|-- THIS SOFTWARE IS PROVIDED BY FREESCALE "AS IS" AND ANY EXPRESSED OR
|-- IMPLIED WARRANTIES, INCLUDING, BUT NOT LIMITED TO, THE IMPLIED WARRANTIES
|-- OF MERCHANTABILITY AND FITNESS FOR A PARTICULAR PURPOSE ARE DISCLAIMED.
|-- IN NO EVENT SHALL FREESCALE OR ITS CONTRIBUTORS BE LIABLE FOR ANY DIRECT,
|-- INDIRECT, INCIDENTAL, SPECIAL, EXEMPLARY, OR CONSEQUENTIAL DAMAGES
|-- (INCLUDING, BUT NOT LIMITED TO, PROCUREMENT OF SUBSTITUTE GOODS OR
|-- SERVICES; LOSS OF USE, DATA, OR PROFITS; OR BUSINESS INTERRUPTION)
|-- HOWEVER CAUSED AND ON ANY THEORY OF LIABILITY, WHETHER IN CONTRACT,
|-- STRICT LIABILITY, OR TORT (INCLUDING NEGLIGENCE OR OTHERWISE) ARISING
|-- IN ANY WAY OUT OF THE USE OF THIS SOFTWARE, EVEN IF ADVISED OF
|-- THE POSSIBILITY OF SUCH DAMAGE.
[IBIS Ver]   5.0
[Comment Char] |_char
[File name]   k60_120_144lqfp_full.ibs
[File Rev]   1.2
[Date]   12/03/2013
[Source]   Freescale, MSG, MCD, Design
[Notes]   IBIS model for K60 microprocessor covers 1.71 - 3.6V range
[Disclaimer]   The model given below represents 144LQFP package on K60 family
[Copyright]   Copyright, Freescale, Inc., 2013
|  Component K60
[Component]   K60
[Manufacturer]  Freescale, Inc.
[Package]
|   typ   min   max
R_pkg   0.13643   0.074674   0.1605
L_pkg   6.219e-9   4.626e-9   7.688e-9
C_pkg   1.386e-12   1.181e-12   1.778e-12
[Pin]   Signal_name   model_name   R_pin   L_pin   C_pin
31   VDDA   POWER
5   VDD   POWER
16   VDD   POWER
43   VDD   POWER
56   VDD   POWER
70   VDD   POWER
94   VDD   POWER
108   VDD   POWER
122   VDD   POWER
135   VDD   POWER
42   VBAT   POWER
21   VOUT33   POWER
22   VREGIN   POWER
36   ADC0SE16   NC   0.14655   6.97e-9   1.242e-12
35   ADC1SE16   NC   0.15005   5.832e-9   1.506e-12
38   DAC0OUT   NC   0.14297   7.255e-9   1.542e-12
39   DAC1OUT   NC   0.14077   7.112e-9   1.559e-12
41   EXTAL32   NC   0.15038   6.782e-9   1.534e-12
28   PGA0DM   NC   0.12334   5.949e-9   1.339e-12
27   PGA0DP   NC   0.12106   5.958e-9   1.357e-12
30   PGA1DM   NC   0.13667   5.32e-9   1.386e-12
29   PGA1DP   NC   0.12773   5.801e-9   1.374e-12
24   PGA2DM   NC   0.11967   5.705e-9   1.317e-12
23   PGA2DP   NC   0.12104   5.634e-9   1.22e-12
26   PGA3DM   NC   0.11999   5.914e-9   1.36e-12
25   PGA3DP   NC   0.11921   5.753e-9   1.321e-12
50   PTA0   io_5vtol   0.14193   6.304e-9   1.346e-12
51   PTA1   io_5vtol   0.14175   6.208e-9   1.311e-12
52   PTA2   io_5vtol   0.14204   6.057e-9   1.268e-12
53   PTA3   io_5vtol   0.14336   5.897e-9   1.296e-12
54   PTA4   io_5vtol   0.14599   5.67e-9   1.273e-12
55   PTA5   io_5vtol   0.15141   5.209e-9   1.264e-12
58   PTA6   io_fast_5vtol   0.14704   5.445e-9   1.181e-12
59   PTA7   io_fast_5vtol   0.14318   5.955e-9   1.316e-12
60   PTA8   io_fast_5vtol   0.14221   6.155e-9   1.403e-12
61   PTA9   io_fast_5vtol   0.14262   6.348e-9   1.365e-12
62   PTA10   io_fast_5vtol   0.14414   6.614e-9   1.329e-12
63   PTA11   io_fast_5vtol   0.14519   6.744e-9   1.315e-12
64   PTA12   io_fast_5vtol   0.14748   6.905e-9   1.497e-12
65   PTA13   io_fast_5vtol   0.15026   7.017e-9   1.504e-12
66   PTA14   io_fast_5vtol   0.15364   7.127e-9   1.546e-12
67   PTA15   io_fast_5vtol   0.15784   7.187e-9   1.595e-12
68   PTA16   io_fast_5vtol   0.15454   6.819e-9   1.507e-12
69   PTA17   io_fast_5vtol   0.16279   6.406e-9   1.497e-12
72   PTA18   io_5vtol   0.16043   6.526e-9   1.251e-12
73   PTA19   io_5vtol   0.15124   7.53e-9   1.238e-12
75   PTA24   io_fast_5vtol   0.14588   7.278e-9   1.672e-12
76   PTA25   io_fast_5vtol   0.14088   7.144e-9   1.574e-12
77   PTA26   io_fast_5vtol   0.13659   6.98e-9   1.557e-12
78   PTA27   io_fast_5vtol   0.13268   6.792e-9   1.527e-12
79   PTA28   io_fast_5vtol   0.12945   6.656e-9   1.373e-12
80   PTA29   io_fast_5vtol   0.12683   6.534e-9   1.39e-12
81   PTB0   io_5vtol   0.12814   6.465e-9   1.315e-12
82   PTB1   io_5vtol   0.12562   6.334e-9   1.282e-12
83   PTB2   io_5vtol   0.12444   6.322e-9   1.332e-12
84   PTB3   io_5vtol   0.12222   6.072e-9   1.188e-12
85   PTB4   io_5vtol   0.12112   5.946e-9   1.208e-12
86   PTB5   io_5vtol   0.12035   5.788e-9   1.261e-12
87   PTB6   io_5vtol   0.1205   5.733e-9   1.251e-12
88   PTB7   io_5vtol   0.12088   5.617e-9   1.323e-12
89   PTB8   io_5vtol   0.12212   5.499e-9   1.25e-12
90   PTB9   io_5vtol   0.12418   5.384e-9   1.259e-12
91   PTB10   io_5vtol   0.12712   5.169e-9   1.236e-12
92   PTB11   io_5vtol   0.13355   4.626e-9   1.199e-12
95   PTB16   io_5vtol   0.1273   5.128e-9   1.245e-12
96   PTB17   io_5vtol   0.12586   5.485e-9   1.249e-12
97   PTB18   io_5vtol   0.12629   5.716e-9   1.269e-12
98   PTB19   io_5vtol   0.12517   6.017e-9   1.309e-12
99   PTB20   io_5vtol   0.12713   6.21e-9   1.298e-12
100   PTB21   io_5vtol   0.12288   6.219e-9   1.481e-12
101   PTB22   io_5vtol   0.12499   6.323e-9   1.434e-12
102   PTB23   io_5vtol   0.12787   6.437e-9   1.509e-12
103   PTC0   io_5vtol   0.1316   6.547e-9   1.606e-12
104   PTC1   io_5vtol   0.1361   6.536e-9   1.477e-12
105   PTC2   io_5vtol   0.14259   6.455e-9   1.623e-12
106   PTC3   io_5vtol   0.1535   5.859e-9   1.717e-12
109   PTC4   io_5vtol   0.15098   7.253e-9   1.234e-12
110   PTC5   io_5vtol   0.14677   7.215e-9   1.63e-12
111   PTC6   io_5vtol   0.14359   7.131e-9   1.778e-12
112   PTC7   io_5vtol   0.14177   7.069e-9   1.644e-12
113   PTC8   io_5vtol   0.14008   6.972e-9   1.555e-12
114   PTC9   io_5vtol   0.1389   6.86e-9   1.458e-12
115   PTC10   io_5vtol   0.13814   6.784e-9   1.455e-12
116   PTC11   io_5vtol   0.14256   6.761e-9   1.421e-12
117   PTC12   io_5vtol   0.14197   6.609e-9   1.445e-12
118   PTC13   io_5vtol   0.14182   6.363e-9   1.338e-12
119   PTC14   io_5vtol   0.14393   6.114e-9   1.299e-12
120   PTC15   io_5vtol   0.15069   5.442e-9   1.29e-12
123   PTC16   io_5vtol   0.15095   5.346e-9   1.331e-12
124   PTC17   io_5vtol   0.14574   5.72e-9   1.254e-12
125   PTC18   io_5vtol   0.14294   5.845e-9   1.28e-12
126   PTC19   io_5vtol   0.1425   5.923e-9   1.323e-12
127   PTD0   io_5vtol   0.14188   5.956e-9   1.311e-12
128   PTD1   io_5vtol   0.14138   5.999e-9   1.364e-12
129   PTD2   io_5vtol   0.14138   6.02e-9   1.256e-12
130   PTD3   io_5vtol   0.14182   6.003e-9   1.269e-12
131   PTD4   io_5vtol   0.14319   5.979e-9   1.332e-12
132   PTD5   io_5vtol   0.14586   5.856e-9   1.384e-12
133   PTD6   io_5vtol   0.1519   5.479e-9   1.337e-12
136   PTD7   io_5vtol   0.095186   5.041e-9   1.478e-12
137   PTD8   io_5vtol   0.14925   6.316e-9   1.492e-12
138   PTD9   io_5vtol   0.14703   6.779e-9   1.509e-12
139   PTD10   io_5vtol   0.14768   7.034e-9   1.474e-12
140   PTD11   io_5vtol   0.14919   7.21e-9   1.461e-12
141   PTD12   io_5vtol   0.14283   7.2e-9   1.515e-12
142   PTD13   io_5vtol   0.1446   7.355e-9   1.608e-12
143   PTD14   io_5vtol   0.14714   7.47e-9   1.636e-12
144   PTD15   io_5vtol   0.15009   7.688e-9   1.254e-12
1   PTE0   io_5vtol   0.1427   7.238e-9   1.207e-12
2   PTE1   io_5vtol   0.13901   6.841e-9   1.585e-12
3   PTE2   io_5vtol   0.1373   6.39e-9   1.599e-12
4   PTE3   io_5vtol   0.14055   5.484e-9   1.55e-12
7   PTE4   io_5vtol   0.13988   5.539e-9   1.415e-12
8   PTE5   io_5vtol   0.13191   5.975e-9   1.399e-12
9   PTE6   io_5vtol   0.12792   6.051e-9   1.458e-12
10   PTE7   io_5vtol   0.128   6.113e-9   1.36e-12
11   PTE8   io_5vtol   0.12596   6.019e-9   1.327e-12
12   PTE9   io_5vtol   0.12369   5.831e-9   1.207e-12
13   PTE10   io_5vtol   0.12287   5.649e-9   1.215e-12
14   PTE11   io_5vtol   0.12314   5.391e-9   1.263e-12
15   PTE12   io_5vtol   0.1281   4.876e-9   1.189e-12
45   PTE24   io_5vtol   0.1605   5.873e-9   1.334e-12
46   PTE25   io_5vtol   0.152   6.343e-9   1.407e-12
47   PTE26   io_5vtol   0.14753   6.409e-9   1.316e-12
48   PTE27   io_5vtol   0.14454   6.387e-9   1.329e-12
49   PTE28   io_5vtol   0.14278   6.348e-9   1.243e-12
74   RESETB   io_5vtol   0.089297   6.831e-9   1.632e-12
20   USB0DM   NC   0.12719   5.235e-9   1.265e-12
19   USB0DP   NC   0.13445   4.892e-9   1.192e-12
32   VREFH   NC   0.14189   5.271e-9   1.448e-12
33   VREFL   NC   0.14543   5.412e-9   1.448e-12
37   VREFOUT   NC   0.14666   7.499e-9   1.204e-12
40   XTAL32   NC   0.15094   7.153e-9   1.538e-12
34   VSSA   GND
6   VSS   GND
17   VSS   GND
18   VSS   GND
44   VSS   GND
57   VSS   GND
71   VSS   GND
93   VSS   GND
107   VSS   GND
121   VSS   GND
134   VSS   GND
|End [Component]
[Component] io80u65dgo6m5vtol
|   Component io80u65dgo6m5vtol
| This component was characterised for following simulation conditions:
| Temperature:
|   - Typ: 25.0C,   - Min: 125.0C,   - Max: -40.0C
| External (pad) voltage:
|   - Typ: 3.3V,   - Min: 1.71V,   - Max: 3.6V
| Internal (core) voltage:
|   - Typ: 1.2V,   - Min: 1.08V,   - Max: 1.32V
[Manufacturer] Freescale Semiconductor
[Package]
| variable   typ   min   max
R_pkg   0.2240   0.2240   0.2240
L_pkg   8.5100nH   8.5100nH   8.5100nH
C_pkg   0.2740pF   0.2740pF   0.2740pF
[Pin]  signal_name   model_name   R_pin   L_pin   C_pin
fpad   pad   io_fast_5vtol
pad   pad   io_5vtol
|vsslv vsslv   iGND
|vddlv vddlv   iPOWER
vdd3v  vdd3v   POWER
vss3v  vss3v   GND
|obe   obe   dummy
|do   do   dummy
[Model Selector] io_fast_5vtol
io_fast_5vtol_dse1_sre0   fast io, full drive mode without slew rate
io_fast_5vtol_dse1_sre1   fast io, full drive mode with slew rate
io_fast_5vtol_dse0_sre0   fast io, low drive mode without slew rate
io_fast_5vtol_dse0_sre1   fast io, low drive mode with slew rate
[Model Selector] io_5vtol
io_5vtol_dse1_sre0   io, full drive mode without slew rate
io_5vtol_dse1_sre1   io, full drive mode with slew rate
io_5vtol_dse0_sre0   io, low drive mode without slew rate
io_5vtol_dse0_sre1   io, low drive mode with slew rate
| Models and submodels in the file (8): io_fast_5vtol_dse1_sre0 (I/O), io_5vtol_dse1_sre0 (I/O), io_fast_5vtol_dse1_sre1 (I/O), io_5vtol_dse1_sre1 (I/O), io_fast_5vtol_dse0_sre0 (I/O), io_5vtol_dse0_sre0 (I/O), io_fast_5vtol_dse0_sre1 (I/O), io_5vtol_dse0_sre1 (I/O)
